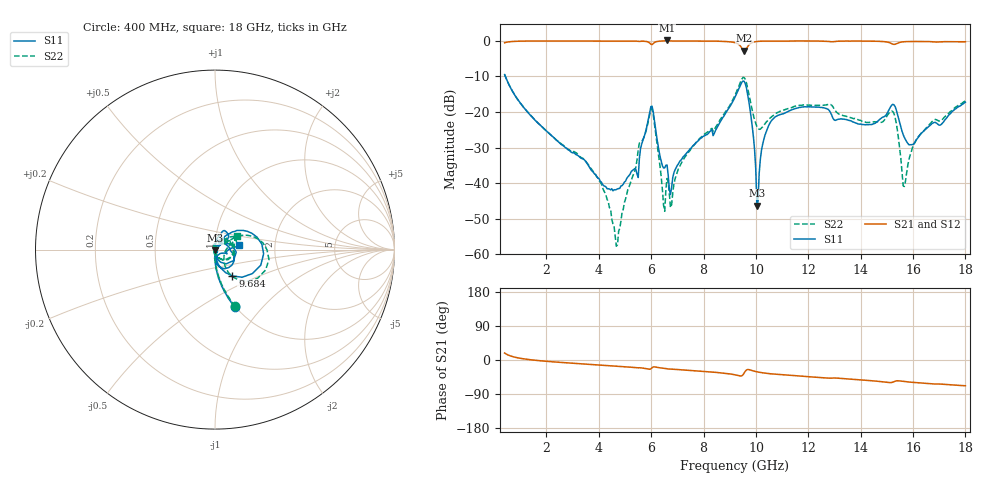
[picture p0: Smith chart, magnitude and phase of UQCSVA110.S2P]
!  Part Number  UQCSVA110  Mounting Orientation: Horizontal
!  Description: Ultra Low ESR Microwave capacitors
!  Application: Coupling, Bypass, Tuning, DC Block
!  Filters, Matching
# GHZ S DB R 50
! Freq  |S11|  S11 Ph  |S21|  S21 Ph  |S12|  S12 Ph  |S22|  S22 Ph
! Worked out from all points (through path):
!   401 points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, 400 MHz to 18 GHz, reference 50 ohm
!   highest |S21| = 0.09 dB at 6.604 GHz (marker M1); lowest = -2.8 dB at 9.552 GHz (marker M2)
!   group delay of S21, straight-line fit = 11.3 ps
!   lowest |S11| = -46.3 dB at 10.04 GHz (marker M3), VSWR 1.01, Z = 50 - j0.482 ohm
!   |S11| at or under -10 dB: 427.7 MHz to end of sweep
!   |S22| runs from -57.7 to -9.5 dB; largest |S21 - S12| = 0.0074
!   S11 on the Smith chart (normalised r, x): 400 MHz: 0.99, -0.71; 9.684 GHz: 1.16, -0.35; 18 GHz: 1.31, +0.07
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0.4  -9.49 -71.0  -0.56 18.4  -0.56 18.5  -9.46 -70.3
3.348  -33.08 -90.1  -0.04 -10.3  -0.03 -10.2  -32.89 -92.2
4.14  -40.33 -72.6  -0.03 -13.8  -0.03 -13.8  -41.28 -101.8
4.712  -41.59 -20.5  -0.03 -16.5  -0.02 -16.4  -57.29 175.4
5.46  -37.52 21.5  -0.12 -20.6  -0.12 -20.5  -33.29 103.8
5.944  -19.95 11.6  -0.65 -24.4  -0.65 -24.3  -20.44 31.2
6.296  -30.90 -74.3  -0.12 -20.3  -0.12 -20.2  -33.03 -75.5
6.428  -35.13 -56.9  -0.06 -21.4  -0.06 -21.3  -41.96 -69.5
6.604  -34.88 -46.3  0.09 -23.0  0.09 -22.9  -38.68 8.6
6.78  -41.09 15.3  -0.06 -24.2  -0.06 -24.1  -46.03 46.0
7.264  -32.32 35.1  -0.05 -26.4  -0.05 -26.3  -32.91 64.8
9.2  -15.81 41.1  -0.53 -39.2  -0.52 -39.1  -15.30 27.6
9.552  -11.39 -18.8  -2.82 -34.3  -2.80 -34.2  -10.35 -22.1
9.684  -15.10 -56.5  -1.62 -25.1  -1.62 -25.2  -13.34 -52.1
10.036  -46.34 -89.8  -0.20 -31.1  -0.20 -31.0  -24.09 -36.3
10.608  -22.29 74.3  -0.10 -36.7  -0.09 -36.6  -21.29 17.2
12.148  -18.57 59.9  -0.06 -44.8  -0.06 -44.6  -18.12 25.7
15.096  -19.19 -18.0  -0.52 -59.5  -0.52 -59.3  -20.21 15.9
15.316  -18.48 -63.3  -0.98 -56.0  -0.96 -55.8  -21.59 -40.3
15.668  -27.12 -79.0  -0.26 -56.8  -0.27 -56.6  -40.93 170.4
16.24  -26.69 -25.7  -0.20 -60.3  -0.19 -60.1  -26.62 76.6
18  -17.26 11.4  -0.28 -68.0  -0.27 -67.8  -16.90 31.8
